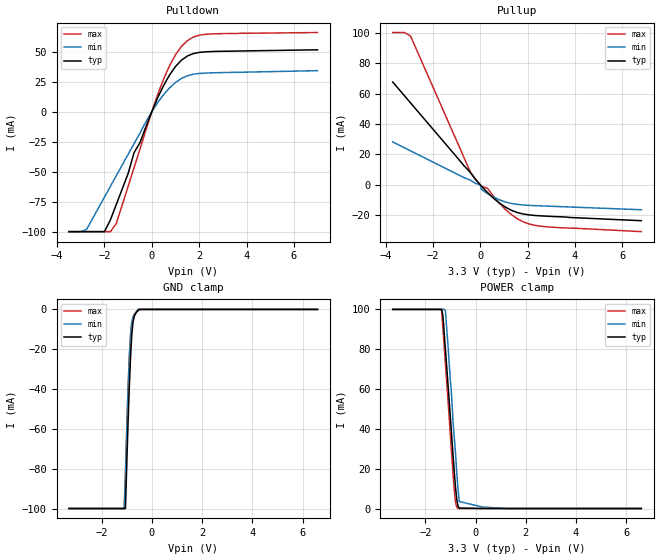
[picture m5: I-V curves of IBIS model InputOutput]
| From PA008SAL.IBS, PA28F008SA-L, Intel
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|**************************Input Output Model*********************************
[Model]   InputOutput
Model_type   I/O
|   for DQ[7:0]
Vinl = 0.8V
Vinh = 2.0V
| Variable   typ   min   max
C_comp   9.61p   NA   11.6p
[Voltage Range]   3.3V   3.0V   3.6V
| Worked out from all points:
|   slope of the pulldown table from 0 to 0.495 V, typ, clamps not added: 22.8 ohm
|   slope of the pullup table from 0 to 0.495 V, typ, clamps not added: 63.2 ohm
|   GND clamp passes 1 mA (typ) near -0.58 V on its own axis
|   POWER clamp passes 1 mA (typ) near -0.69 V on its own axis
[Pulldown]
| [Pullup] and [Pulldown] IV curves include only the current through
| the channels of output driver transistors when outputs are enabled
| with OE# = VIL.  Although the output driver transistors have np and
| pn diodes inherently created by CMOS IC fabrication between the
| drain and bulk of n-channel and p-channel CMOS transistors,
| the current through these junction diodes is not included in
| [Pullup] or [Pulldown].  Instead that drain/bulk diode current is
| included in the [POWER_clamp] or [GND_clamp] sections, which are
| not dependent on the state of OE# or output data value.
|Voltage  I(typ)   I(min)   I(max)
-3.5V     -100mA     -100mA     -100mA
-2.75V    -100mA     -97.98mA   -100mA
-2V       -100mA     -71.2mA    -100mA
-1.75V    -90.2mA    -62.28mA   -100mA
-1.5V     -77.3mA    -53.35mA   -93.26mA
-1V       -51.5mA    -35.5mA    -62.16mA
-750mV    -34.15mA   -26.58mA   -46.61mA
500mV     21.94mA    14.3mA     27.3mA
1V        37.7mA     24.38mA    47.5mA
1.5V      46.44mA    29.97mA    59.25mA
2.5V      50.13mA    32.38mA    64.82mA
7V        51.6mA     34.2mA     66mA
[GND_clamp]
| [POWER_clamp] and [GND_clamp] IV curves describe ESD protection
| circuits PLUS some np and pn diodes which exist between the
| drain and bulk of n-channel and p-channel CMOS transistors.
| These drain/bulk diodes are inherent in CMOS IC fabrication,
| and are visible on the node of the I/O pin at all times.
| Even the drain/bulk diodes of output driver [Pullup] and [Powerdown]
| transistors are included in [POWER_clamp] or [GND_clamp], because
| these diodes contribute to I/O pin current even when the
| chip outputs are tristated by OE# = VIH.
| For example, when V forced on the I/O pin is large, we are
| forward biasing the pn diode at the drain/bulk interface in the
| p-channel pullup transistor.  Similarly, when V forced on the
| I/O pin is sufficiently negative with respect to the substrate
| ground, we are forward biasing the np diode at the drain/bulk
| interface in the n-channel pulldown transistor.  The effects
| of these diodes are included in [POWER_clamp] or [GND_clamp].
|Voltage  I(typ)   I(min)   I(max)
-3.3V     -100mA     -100mA     -100mA
-1.1V     -100mA     -100mA     -100mA
-1.05V    -100mA     -83.54mA   -82.54mA
-1V       -78.71mA   -61.79mA   -60.79mA
-950mV    -58.42mA   -42mA      -41.03mA
-900mV    -39.92mA   -25.35mA   -24.35mA
-850mV    -24.72mA   -14mA      -12.89mA
-800mV    -13.16mA   -6.667mA   -6.654mA
-750mV    -6.532mA   -4.159mA   -4.069mA
-700mV    -3.516mA   -2.6mA     -2.683mA
-550mV    -696.6uA   0A         0A
6.6V      0A         0A         0A
[Pullup]
| (Voltages for [Pullup] and [POWER_clamp] are specified with
| negative respect to Vcc.  Reference the IBIS documentation
| for more information regarding Vtable = Vcc - Voutput.
| This method keeps -Vds constant for the values in all three
| columns across a line of the table.
| [Pullup] and [Pulldown] IV curves include only the current through
| the channels of output driver transistors when outputs are enabled
| with OE# = VIL.  Although the output driver transistors have np and
| pn diodes inherently created by CMOS IC fabrication between the
| drain and bulk of n-channel and p-channel CMOS transistors,
| the current through these junction diodes is not included in
| [Pullup] or [Pulldown].  Instead that drain/bulk diode current is
| included in the [POWER_clamp] or [GND_clamp] sections, which are
| not dependent on the state of OE# or output data value.
|Voltage  I(typ)   I(min)   I(max)
-3.7V     67.54mA    28.26mA    100mA
-3.2V     58.44mA    24.36mA    100mA
-2.95V    53.89mA    22.41mA    97.81mA
-450mV    8.674mA    3.388mA    9.383mA
0V        0A         0A         0A
50mV      -851.5uA   -3.019mA   -1mA
300mV     -4.966mA   -5.654mA   -2.153mA
550mV     -8.646mA   -7.891mA   -7.271mA
1.3V      -16.53mA   -12.11mA   -19.29mA
1.8V      -19.03mA   -13.13mA   -24.13mA
2.55V     -20.28mA   -13.73mA   -27.07mA
6.8V      -23.46mA   -16.28mA   -30.64mA
[POWER_clamp]
| (Voltages for [Pullup] and [POWER_clamp] are specified with
| negative respect to Vcc.  Reference the IBIS documentation
| for more information regarding Vtable = Vcc - Voutput.
| This method keeps -Vds constant for the values in all three
| columns across a line of the table.
| [POWER_clamp] and [GND_clamp] IV curves describe ESD protection
| circuits PLUS some np and pn diodes which exist between the
| drain and bulk of n-channel and p-channel CMOS transistors.
| These drain/bulk diodes are inherent in CMOS IC fabrication,
| and are visible on the node of the I/O pin at all times.
| Even the drain/bulk diodes of output driver [Pullup] and [Powerdown]
| transistors are included in [POWER_clamp] or [GND_clamp], because
| these diodes contribute to I/O pin current even when the
| chip outputs are tristated by OE# = VIH.
| For example, when V forced on the I/O pin is large, we are
| forward biasing the pn diode at the drain/bulk interface in the
| p-channel pullup transistor.  Similarly, when V forced on the
| I/O pin is sufficiently negative with respect to the substrate
| ground, we are forward biasing the np diode at the drain/bulk
| interface in the n-channel pulldown transistor.  The effects
| of these diodes are included in [POWER_clamp] or [GND_clamp].
|Voltage  I(typ)   I(min)   I(max)
-3.3V     100mA      100mA      100mA
-1.35V    100mA      100mA      99.18mA
-1.3V     96.69mA    100mA      90.34mA
-1.2V     79.76mA    99.28mA    72.59mA
-950mV    36.17mA    56mA       26.92mA
-900mV    27.31mA    44mA       17.8mA
-850mV    18.68mA    36mA       9.459mA
-800mV    10.82mA    28mA       3.42mA
-700mV    1.279mA    9.6mA      0A
-650mV    227.9uA    3.5mA      0A
300mV     0A         700uA      0A
6.6V      0A         0A         0A
[Ramp]
| The DQ Ramp information is not provided at this time for the
| device but will be available in the future.  The table below
| is for the compatibility with some IBIS parsers.
| Variable   typ   min   max
 dV/dt_r   0V/0ns   0V/0ns   0V/0ns
 dV/dt_f   0V/0ns   0V/0ns   0V/0ns
